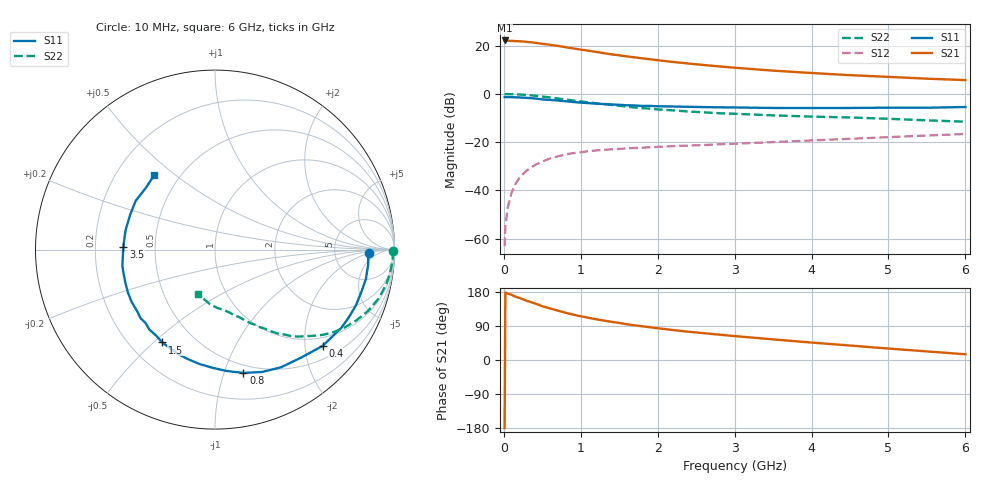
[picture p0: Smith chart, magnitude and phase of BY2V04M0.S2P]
! SIEMENS Small Signal Semiconductors
! BFY420
! Si NPN RF SIEGET Grounded Emitter Transistor in MICRO-X
! VCE = 2 V  IC = 4 mA
! Common Emitter S-Parameters:  October  1996
# GHz  S  MA  R  50
!  f  S11  S21  S12  S22
! GHz  MAG  ANG  MAG  ANG  MAG  ANG  MAG  ANG
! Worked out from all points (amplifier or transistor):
!   36 points, 10 MHz to 6 GHz, reference 50 ohm
!   highest |S21| = 22.1 dB at 10 MHz (marker M1)
!   |S21| within 3 dB of that: start of sweep to 844 MHz
!   unconditionally stable (mu >= 1): 3.338 GHz to end of sweep
!   at 250 MHz: K = 0.10, MSG = 27.5 dB, |S12| = -33.2 dB
!   at 1.4 GHz: K = 0.46, MSG = 19.7 dB, |S12| = -23.0 dB
!   at 6 GHz: K = 1.17, MAG = 8.7 dB, |S12| = -16.6 dB
!   S11 on the Smith chart (normalised r, x): 10 MHz: 13, -2; 400 MHz: 0.79, -2.40; 800 MHz: 0.43, -1.16; 1.5 GHz: 0.33, -0.53; 3.5 GHz: 0.32, +0.01; 6 GHz: 0.36, +0.42
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0.01  0.8597 -1.2  12.8 -180.0  0.0007 107.4  0.9933 -0.5
0.02  0.8545 -2.3  12.74 177.9  0.0018 89.8  0.9895 -1.1
0.05  0.8574 -5.3  12.55 175.3  0.0044 85.2  0.9918 -2.9
0.1  0.8568 -11.0  12.55 172.2  0.0089 85.2  0.987 -5.8
0.15  0.8486 -16.3  12.4 167.2  0.0135 79.4  0.9812 -8.6
0.25  0.8356 -26.9  12.18 159.9  0.0219 74.8  0.961 -14.2
0.3  0.8278 -31.8  11.94 156.1  0.0261 73.1  0.95 -16.9
0.4  0.8048 -41.8  11.53 149.6  0.0333 67.7  0.9173 -22.0
0.5  0.7702 -51.2  10.91 141.9  0.0398 63.3  0.8809 -26.6
0.6  0.7519 -60.7  10.42 136.2  0.0458 58.9  0.8435 -30.9
0.8  0.7049 -77.0  9.31 124.8  0.0555 51.3  0.7675 -38.2
0.9  0.6799 -84.4  8.761 119.8  0.0593 48.9  0.7303 -41.1
1.1  0.6429 -97.9  7.866 111.5  0.065 44.1  0.6671 -46.6
1.3  0.6171 -109.4  6.994 104.1  0.0694 40.5  0.6116 -50.7
1.5  0.5946 -119.6  6.303 97.8  0.0725 37.6  0.5655 -54.5
1.8  0.563 -133.4  5.449 88.9  0.0769 34.8  0.5082 -59.0
2.2  0.5484 -147.9  4.586 79.1  0.0828 32.3  0.4562 -64.2
2.8  0.5267 -165.2  3.714 66.9  0.0902 30.3  0.3969 -70.7
3.5  0.5112 178.2  3.035 54.4  0.1004 28.6  0.3591 -77.2
4.5  0.5111 157.7  2.446 38.2  0.1173 25.4  0.3247 -87.9
5.5  0.5167 138.0  2.067 22.7  0.1374 21.0  0.2831 -102.4
6  0.5351 129.5  1.934 15.1  0.1476 18.1  0.2659 -111.4
